PROGRAM MAIN
VAR
	RegistrationSensor				: BOOL;
END_VAR

//***************************************************************************************************************
//  The sample uses a rotational knife TO cut sheets OF a defined length. FOR THIS purpose the circumference
//  speed must be synchronized with the web while cutting a sheet. The rotation knife must the accelerator or
//  deceleration since the circumference of the knife is different from the sheet length. Registration marks are
//  used to synchronize with the product. The knife is continuously adjusted to compensate small differences
//  caused by temperature or stretching.
//  An electronic cam table is used to synchronize the rotational knife with the material. The cam table is a
//  normalized cam table defined with a length of 360°. The tool moves over a full turn while the cam table is
//  executed and the cut position is defined as 0°. The circumference speed is synchronous from 270° to 30°.
//  The range from 30° to 270° is used to adjust the operation to the actual distance of registration marks.

(* update the axis status at the beginning of each cycle *)

//***************************************************************************************************************
//  The sample uses a rotational knife TO cut sheets OF a defined length. FOR THIS purpose the circumference
//  speed must be synchronized with the web while cutting a sheet. The rotation knife must the accelerator or
//  deceleration since the circumference of the knife is different from the sheet length. Registration marks are
//  used to synchronize with the product. The knife is continuously adjusted to compensate small differences
//  caused by temperature or stretching.
//  An electronic cam table is used to synchronize the rotational knife with the material. The cam table is a
//  normalized cam table defined with a length of 360°. The tool moves over a full turn while the cam table is
//  executed and the cut position is defined as 0°. The circumference speed is synchronous from 270° to 30°.
//  The range from 30° to 270° is used to adjust the operation to the actual distance of registration marks.




WebTransport();
VirtualWeb();
RotaryKnife();

(* call simulation of a registration mark *)
//RegistrationMarkSimulation( ProductLength:=PRODUCTLENGTH, Axis:=WebTransport );
//RegistrationSensor := RegistrationMarkSimulation.RegistrationSignal;

(* rotary knife state machine *)
RotaryKnifeApplication( RegistrationSensor:=RegistrationSensor );

END_PROGRAM
